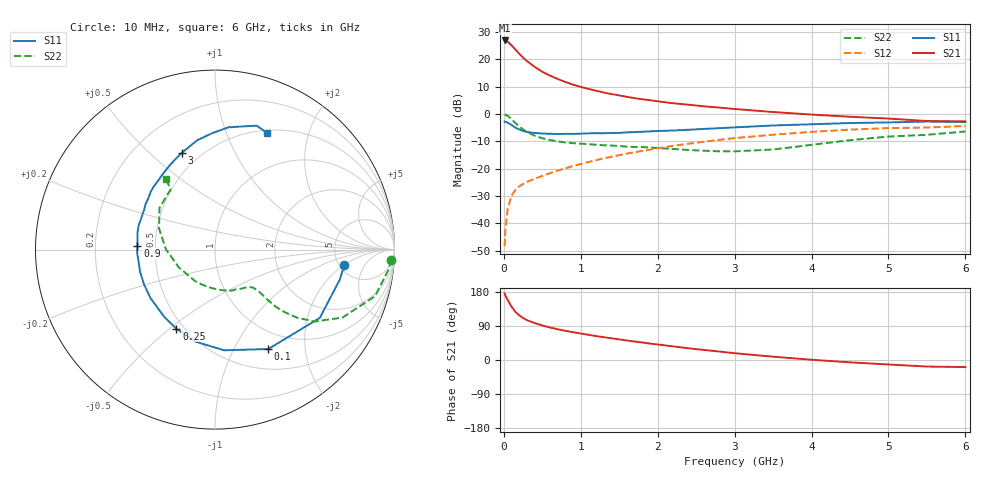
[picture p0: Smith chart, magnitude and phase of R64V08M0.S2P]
! SIEMENS Small Signal Semiconductors
! BFR193
! Si NPN RF Bipolar Junction Transistor in SOT23
! VCE = 4 V  IC = 8 mA
! Common Emitter S-Parameters:  May  1996
# GHz  S  MA  R  50
!  f  S11  S21  S12  S22
! GHz  MAG  ANG  MAG  ANG  MAG  ANG  MAG  ANG
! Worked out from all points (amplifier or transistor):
!   36 points, 10 MHz to 6 GHz, reference 50 ohm
!   highest |S21| = 27.0 dB at 10 MHz (marker M1)
!   |S21| within 3 dB of that: start of sweep to 139.7 MHz
!   unconditionally stable (mu >= 1): 780 MHz to 1.958 GHz
!   at 250 MHz: K = 0.57, MSG = 23.2 dB, |S12| = -25.6 dB
!   at 1.4 GHz: K = 1.05, MAG = 10.1 dB, |S12| = -15.7 dB
!   at 6 GHz: K = 0.95, MSG = 0.8 dB, |S12| = -4.4 dB
!   lowest NFmin = 1.25 dB at 450 MHz
!   S11 on the Smith chart (normalised r, x): 10 MHz: 5.49, -2.04; 100 MHz: 0.76, -1.38; 250 MHz: 0.45, -0.53; 900 MHz: 0.40, +0.02; 3 GHz: 0.40, +0.64; 6 GHz: 0.53, +1.40
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0.01  0.725 -7.0  22.29 175.6  0.0038 85.3  0.9843 -3.3
0.02  0.7149 -13.6  22.28 170.8  0.0075 84.8  0.9728 -6.7
0.05  0.697 -33.1  21.16 158.3  0.0182 74.1  0.9287 -16.2
0.1  0.6285 -61.8  18.22 140.8  0.0318 64.7  0.8057 -28.0
0.15  0.5633 -84.8  15.21 127.0  0.0409 57.4  0.6851 -35.8
0.2  0.5243 -101.9  12.75 118.0  0.0475 54.6  0.5939 -39.7
0.25  0.4903 -116.0  10.82 110.7  0.0523 53.1  0.5222 -41.9
0.3  0.4698 -126.9  9.372 105.2  0.0572 53.3  0.4688 -43.2
0.4  0.4498 -143.0  7.32 97.5  0.0653 54.3  0.4018 -43.7
0.5  0.4401 -154.3  5.954 91.1  0.0736 55.7  0.3607 -43.6
0.6  0.4353 -163.8  5.057 85.8  0.0826 57.3  0.3337 -43.7
0.7  0.4306 -171.3  4.394 81.1  0.092 58.6  0.3157 -44.3
0.9  0.4325 177.2  3.455 73.3  0.112 60.2  0.2931 -45.7
1.1  0.4425 167.1  2.892 66.5  0.1322 61.2  0.2806 -49.0
1.3  0.4456 158.3  2.48 60.2  0.1545 61.3  0.2681 -52.6
1.6  0.4618 147.2  2.063 51.4  0.1883 60.0  0.2531 -60.4
2.2  0.4991 129.1  1.577 35.9  0.2613 55.3  0.2297 -80.4
3  0.5701 109.0  1.238 17.9  0.3623 45.2  0.2076 -122.1
3.5  0.6174 99.2  1.089 8.7  0.4185 37.6  0.2241 -153.5
4.5  0.6852 83.8  0.892 -6.2  0.5182 22.2  0.3327 159.5
5.5  0.7283 71.4  0.746 -17.3  0.5663 6.2  0.4168 126.3
6  0.7121 65.9  0.735 -18.7  0.6051 1.5  0.4792 124.9
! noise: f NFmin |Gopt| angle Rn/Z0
0.45  1.25  0.23  133  0.12
0.9  1.3  0.35  156  0.11
1.8  2  0.55  -155  0.13
